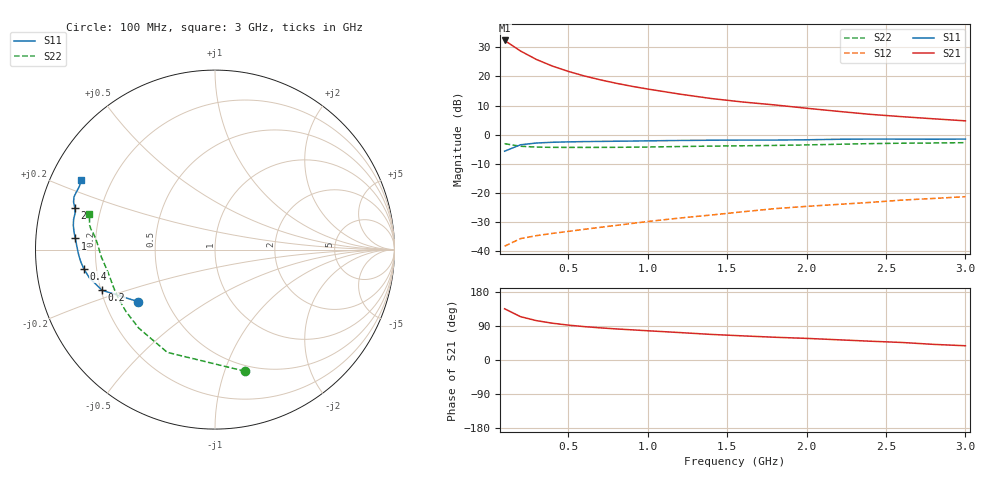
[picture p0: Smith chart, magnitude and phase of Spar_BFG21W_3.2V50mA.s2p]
! Filename: 3_250bfg21.001
! Title: BFG21W
! Bias: Vce=3.2V; Ic=50mA
! Company: NXP Semiconductors NL
! User: Quality&Reliability T&D
! Measure time: 10 Nov 1999 / 11:42:27
#  MHz  S  MA  R 50
! Freq  S11  S21  S12  S22  :
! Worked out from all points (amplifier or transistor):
!   20 points, 100 MHz to 3 GHz, reference 50 ohm
!   highest |S21| = 32.3 dB at 100 MHz (marker M1)
!   |S21| within 3 dB of that: start of sweep to 182.7 MHz
!   unconditionally stable (mu >= 1): 872.9 MHz to end of sweep
!   at 400 MHz: K = 0.69, MSG = 28.8 dB, |S12| = -33.9 dB
!   at 1.2 GHz: K = 1.06, MAG = 19.8 dB, |S12| = -28.7 dB
!   at 3 GHz: K = 1.06, MAG = 11.5 dB, |S12| = -21.3 dB
!   S11 on the Smith chart (normalised r, x): 100 MHz: 0.34, -0.27; 200 MHz: 0.20, -0.17; 400 MHz: 0.15, -0.07; 1 GHz: 0.12, +0.04; 2 GHz: 0.10, +0.14; 3 GHz: 0.09, +0.24
100  0.5189 -146.1  41.44 135.2  0.01212 50.9  0.6979 -76.2
200  0.6689 -160.2  27.29 114.4  0.01634 42.3  0.6313 -114.9
300  0.7172 -167.3  19.55 103.9  0.01837 41.7  0.6098 -134.2
400  0.7384 -171.6  15.07 97.1  0.02007 43.8  0.6041 -145.3
500  0.7504 -174.7  12.21 92.1  0.02172 46.6  0.6028 -152.4
600  0.7584 -177.2  10.2 88.1  0.02356 49.4  0.6028 -157.4
700  0.7641 -179.3  8.761 84.9  0.0255 52.2  0.6033 -161.2
800  0.7694 178.8  7.642 82.0  0.02752 54.7  0.6049 -164.4
900  0.7748 177.1  6.767 79.6  0.02971 57.4  0.6081 -167.1
1000  0.7813 175.4  6.072 77.2  0.03214 59.3  0.6124 -169.4
1200  0.7927 172.6  4.974 72.5  0.03682 62.3  0.6237 -173.3
1400  0.8009 170.3  4.17 67.5  0.04157 64.4  0.6349 -176.4
1600  0.8055 167.9  3.629 63.7  0.04724 66.1  0.6427 -179.1
1800  0.8055 165.5  3.235 60.0  0.05347 67.3  0.6521 178.1
2000  0.8147 163.4  2.838 57.1  0.05851 68.7  0.6654 175.1
2200  0.8315 161.4  2.508 53.4  0.06326 69.3  0.6823 172.6
2400  0.8387 159.5  2.23 49.6  0.06838 69.0  0.7 170.7
2600  0.8367 157.6  2.034 46.3  0.07496 68.5  0.7116 169.0
2800  0.8336 155.2  1.869 41.2  0.08002 67.2  0.7179 166.9
3000  0.8387 152.6  1.724 37.6  0.0859 66.6  0.727 164.3
